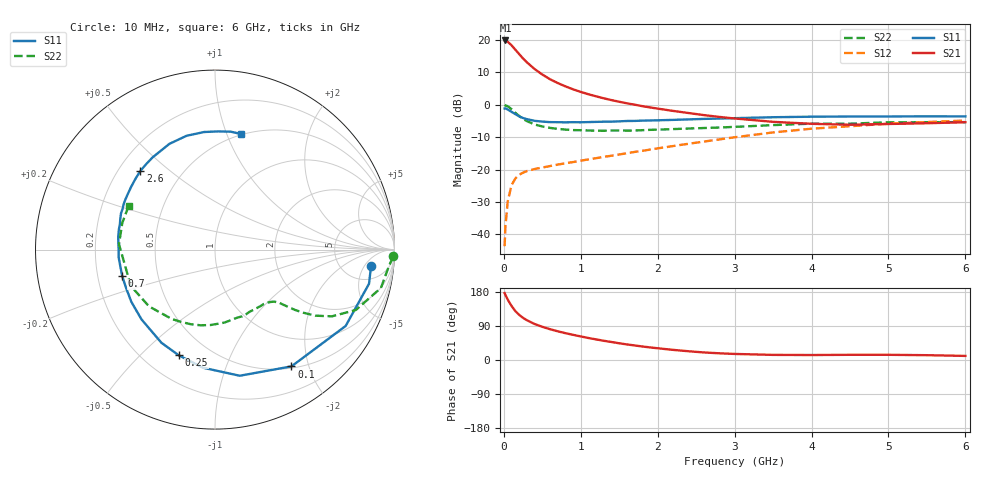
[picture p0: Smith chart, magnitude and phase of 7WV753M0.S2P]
! Infineon Technologies  Discrete & RF Semiconductors
! BFS17W
! Si NPN RF Bipolar Junction Transistor in SOT323
! VCE = 0.75 V  IC = 3 mA
! Common Emitter S-Parameters:  August  1999
# GHz  S  MA  R  50
!  f  S11  S21  S12  S22
! GHz  MAG  ANG  MAG  ANG  MAG  ANG  MAG  ANG
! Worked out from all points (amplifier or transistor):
!   36 points, 10 MHz to 6 GHz, reference 50 ohm
!   highest |S21| = 19.8 dB at 20 MHz (marker M1)
!   |S21| within 3 dB of that: start of sweep to 155.3 MHz
!   unconditionally stable (mu >= 1): 615.2 MHz to end of sweep
!   at 250 MHz: K = 0.48, MSG = 17.6 dB, |S12| = -20.9 dB
!   at 1.4 GHz: K = 1.40, MAG = 4.8 dB, |S12| = -15.7 dB
!   at 6 GHz: K = 1.14, MAG = -2.5 dB, |S12| = -4.9 dB
!   S11 on the Smith chart (normalised r, x): 10 MHz: 9, -7; 100 MHz: 0.52, -1.73; 250 MHz: 0.34, -0.66; 700 MHz: 0.31, -0.13; 2.6 GHz: 0.29, +0.40; 6 GHz: 0.49, +1.12
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0.01  0.8743 -6.1  9.781 176.5  0.0066 86.4  0.9935 -2.2
0.02  0.879 -12.5  9.788 171.8  0.013 86.1  0.9741 -5.3
0.05  0.8432 -30.3  9.361 159.6  0.0321 74.4  0.9489 -13.0
0.1  0.7777 -56.8  8.246 142.7  0.0576 61.1  0.8539 -23.2
0.15  0.7162 -78.9  7.045 129.0  0.0729 51.4  0.7503 -29.7
0.2  0.6615 -95.8  6.018 119.0  0.0835 45.8  0.6687 -33.4
0.25  0.6226 -108.9  5.155 111.2  0.0897 41.2  0.6032 -35.6
0.3  0.5988 -119.9  4.494 104.9  0.0949 39.6  0.559 -37.0
0.4  0.5647 -136.5  3.549 95.0  0.102 37.3  0.4958 -38.7
0.5  0.5495 -148.0  2.918 87.6  0.1076 37.4  0.4624 -39.7
0.6  0.5395 -156.8  2.474 81.3  0.1133 37.9  0.4393 -41.3
0.7  0.5379 -164.0  2.16 75.8  0.1193 39.2  0.4247 -43.4
0.9  0.5383 -175.2  1.727 66.4  0.1306 41.3  0.4064 -48.3
1.1  0.5401 175.8  1.45 58.0  0.1438 43.5  0.4006 -54.3
1.3  0.5473 168.1  1.255 50.7  0.1571 45.3  0.3964 -61.1
1.6  0.5613 158.9  1.051 41.1  0.1786 47.9  0.3989 -71.5
2.2  0.5838 143.1  0.803 26.7  0.2305 50.8  0.421 -93.4
2.6  0.6044 133.4  0.692 19.9  0.2704 50.7  0.4372 -108.1
3.5  0.6417 113.3  0.545 13.5  0.3741 45.7  0.485 -139.3
4.5  0.6579 95.3  0.491 13.7  0.4663 34.8  0.5106 -171.5
5.5  0.6628 82.4  0.518 12.7  0.5404 24.5  0.5375 163.9
6  0.6602 77.5  0.538 10.8  0.5706 19.4  0.5393 153.1
